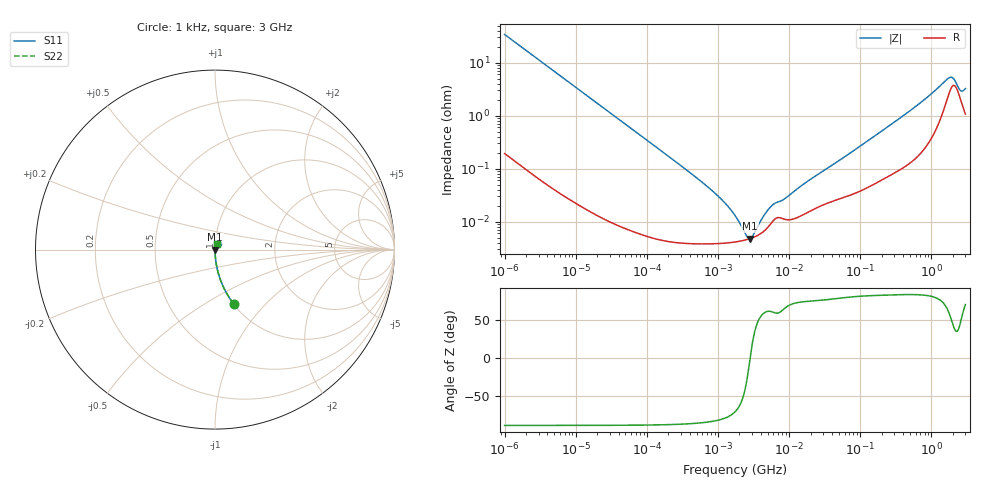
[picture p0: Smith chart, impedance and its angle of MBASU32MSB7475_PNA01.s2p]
! MBASU32MSB7475_PNA01  S-PARAMETER MODEL  ( Standard Model )
! Model Generated by TAIYO YUDEN Corporation (http://www.ty-top.com)
! Version 1.0
! TAIYO YUDEN Control No. 220601
! Copyright(c) 2015 TAIYO YUDEN CO.,LTD. All Rights Reserved.
! Product Description (link to TY-COMPAS)
! https://ds.yuden.co.jp/TYCOMPAS/or/detail?pn=MBASU32MSB7475KPNA01&u=M
! Products Name : Multilayer Ceramic Capacitors
! Characteristics :
!  Capacitance : 4.7 [uF] , Rated Voltage : 50 [V] , TCC : X7R
!  Case Size : 3.2 x 2.5 / 0.126 x 0.098 [mm/inch] , Thickness : 2.5 / 0.098 [mm/inch]
!  (Conditions: Temperature = 25 [degC] , DC Bias Voltage = 0 [V])
! External Node Assignments :
!  1  o---| |---o  2
! GND o---------o GND
! Frequency Range : 1kHz  -  3GHz  [ 401 STEP ]
# MHZ S RI R 50
! Freq[MHz].  S11 Real  S11 Imag  S21 Real  S21 Imag  S12 Real  S12 Imag  S22 Real  S22 Imag
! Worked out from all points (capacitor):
!   401 points, 1 kHz to 3 GHz, reference 50 ohm
!   read as one part in series: C = 4.69 uF near 1.077 kHz
!   lowest |Z| = 4.78 mohm at 2.812 MHz (marker M1)
!   series resonance near 2.828 MHz, so ESL is about 670 pH
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0.001  0.1043 -0.3028  0.8957 0.3028  0.8957 0.3028  0.1043 -0.3028
0.001685  0.04 -0.1931  0.96 0.1931  0.96 0.1931  0.04 -0.1931
0.00306  0.0128 -0.1096  0.9872 0.1096  0.9872 0.1096  0.0128 -0.1096
0.01216  0.000977 -0.0281  0.999 0.0281  0.999 0.0281  0.000977 -0.0281
0.147855  5.09e-05 -0.00233  0.9999 0.00233  0.9999 0.00233  5.09e-05 -0.00233
0.821683  3.83e-05 -0.000384  1 0.000384  1 0.000384  3.83e-05 -0.000384
1.285341  3.94e-05 -0.000213  1 0.000213  1 0.000213  3.94e-05 -0.000213
1.732051  4.12e-05 -0.000124  1 0.000124  1 0.000124  4.12e-05 -0.000124
1.937042  4.22e-05 -9.42e-05  1 9.42e-05  1 9.42e-05  4.22e-05 -9.42e-05
2.087011  4.3e-05 -7.5e-05  1 7.5e-05  1 7.5e-05  4.3e-05 -7.5e-05
2.812335  4.78e-05 -1.36e-06  1 1.36e-06  1 1.36e-06  4.78e-05 -1.36e-06
3.789741  5.71e-05 7.22e-05  0.9999 -7.22e-05  0.9999 -7.22e-05  5.71e-05 7.22e-05
5.928204  0.000102 0.000183  0.9999 -0.000183  0.9999 -0.000183  0.000102 0.000183
8.606987  0.000111 0.000244  0.9999 -0.000244  0.9999 -0.000244  0.000111 0.000244
21.06097  0.000165 0.000639  0.9998 -0.000639  0.9998 -0.000639  0.000165 0.000639
256.0921  0.00077 0.0064  0.9992 -0.0064  0.9992 -0.0064  0.00077 0.0064
727.4359  0.00236 0.018  0.9976 -0.018  0.9976 -0.018  0.00236 0.018
1714.862  0.0244 0.0424  0.9756 -0.0424  0.9756 -0.0424  0.0244 0.0424
1847.629  0.0314 0.0403  0.9686 -0.0403  0.9686 -0.0403  0.0314 0.0403
1990.675  0.0364 0.0339  0.9636 -0.0339  0.9636 -0.0339  0.0364 0.0339
2584.342  0.0196 0.0211  0.9804 -0.0211  0.9804 -0.0211  0.0196 0.0211
3000  0.0114 0.0298  0.9886 -0.0298  0.9886 -0.0298  0.0114 0.0298
